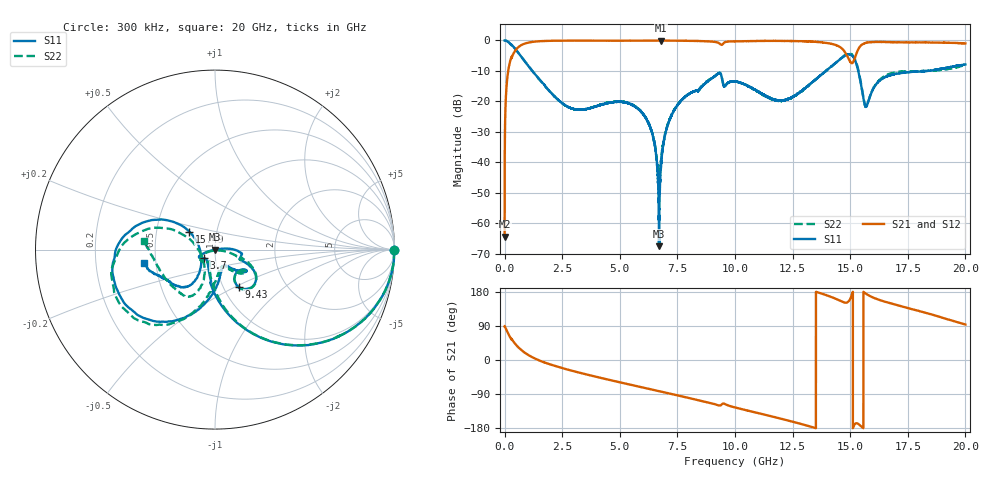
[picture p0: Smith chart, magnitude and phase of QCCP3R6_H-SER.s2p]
!{QCCP3R6}
!Johanson Technology Inc.
!www.johansontechnology.com
!Test Board Conditions:
!Substrate Type  RO4350B
!Substrate Thickness  20 mil
!Substrate Dk  3.66
!TL Type: GCPW
!TL Trace Width  36 mil
!TL Gap  12 mil
!Electrode orientation  Horizontal
!DUT TOPOLOGY	SERIES
!Mounting Pad LxW  26x36 mil
! Created Sat Jan  9 18:29:17 2021
# hz S ma R 50
! 2 Port Network Data from SP1.SP block
! freq  magS11  angS11  magS21  angS21  magS12  angS12  magS22  angS22
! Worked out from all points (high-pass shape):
!   20001 points, 300 kHz to 20 GHz, reference 50 ohm
!   highest |S21| = -0.03 dB at 6.804 GHz (marker M1); lowest = -64.4 dB at 300 kHz (marker M2)
!   |S21| within 3 dB of the highest: 492.3 MHz to 14.69 GHz (14.2 GHz wide, 187 % of centre); 15.34 GHz to end of sweep
!   lowest |S11| = -67.5 dB at 6.707 GHz (marker M3), VSWR 1.00, Z = 50 - j0.028 ohm
!   |S11| at or under -10 dB: 1.205 GHz to 13.94 GHz (12.74 GHz wide, 168 % of centre); 15.35 GHz to 18.36 GHz (3.012 GHz wide, 17.9 % of centre); 18.36312 GHz to 18.36447 GHz (1.344 MHz wide, 0.00732 % of centre)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
!   |S22| runs from -46.0 to 0.0 dB; largest |S21 - S12| = 0.017
!   S11 on the Smith chart (normalised r, x): 300 kHz: open; 3.7 GHz: 0.88, -0.09; 9.43 GHz: 1.18, -0.52; 15.49 GHz: 0.74, +0.15; 20 GHz: 0.43, -0.08
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300000  0.9987 -0.2  0.0006049 88.9  0.0006652 89.9  0.9991 -0.2
1.243e8  0.9649 -16.1  0.2564 73.6  0.2573 73.6  0.9653 -16.1
4.263e8  0.7553 -44.4  0.6489 45.2  0.6506 45.3  0.7548 -44.3
1.3003e9  0.285 -86.2  0.9563 4.4  0.9551 4.4  0.2855 -84.5
3.3343e9  0.07325 -134.7  0.9934 -34.7  0.9927 -34.8  0.07351 -114.3
3.7003e9  0.07723 -141.2  0.9929 -40.3  0.993 -40.3  0.07756 -118.6
5.9313e9  0.06725 -161.5  0.993 -71.6  0.9933 -71.6  0.06767 -158.0
6.4403e9  0.02682 -165.5  0.9944 -78.6  0.9951 -78.6  0.02675 -160.2
6.6673e9  0.003883 -166.1  0.9952 -81.7  0.9949 -81.7  0.006778 -122.0
6.7073e9  0.0004231 -41.5  0.9943 -82.3  0.995 -82.2  0.005257 -81.7
6.8043e9  0.01048 9.8  0.9962 -83.6  0.9944 -83.6  0.01254 -24.5
7.0043e9  0.03285 7.1  0.9932 -86.4  0.9944 -86.4  0.03335 -8.9
7.4603e9  0.08212 3.2  0.9925 -92.7  0.9902 -92.7  0.08333 -12.1
9.4303e9  0.2456 -57.7  0.8478 -116.8  0.8503 -116.8  0.2483 -58.2
1.00003e10  0.2131 -35.2  0.9671 -125.1  0.9666 -125.1  0.2118 -37.8
1.19463e10  0.1041 -62.4  0.9825 -154.2  0.9848 -154.1  0.1023 -66.8
1.33343e10  0.2038 -87.6  0.9571 -176.8  0.9612 -176.8  0.2016 -92.8
1.49713e10  0.587 -161.0  0.4689 158.0  0.4651 157.7  0.6124 -155.1
1.54853e10  0.1752 145.1  0.8383 -175.6  0.8363 -175.8  0.1823 155.6
1.57093e10  0.0833 -159.9  0.9182 174.0  0.9197 173.9  0.08494 -147.8
1.66673e10  0.263 -128.1  0.9381 151.0  0.9336 150.8  0.28 -115.5
2e10  0.4037 -168.9  0.8926 93.7  0.8839 93.4  0.3974 173.1
